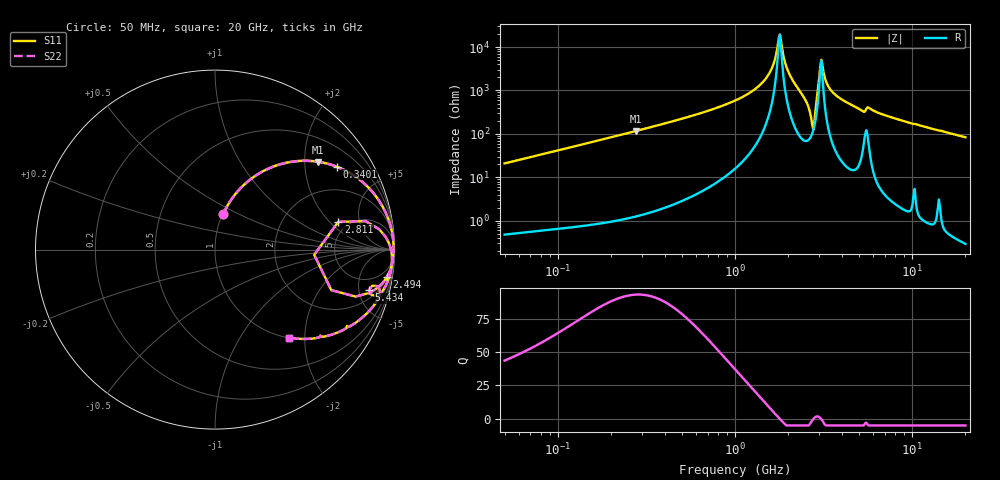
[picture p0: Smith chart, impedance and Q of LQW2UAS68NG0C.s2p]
!Murata Part Number: LQW2UAS68NG0C
!These Parameters are Measured in Series Mode Connection
!  o--[Z]--o
!Port1  Port2
!  o-------o
!Freq. Start=50[MHz] Stop=20[GHz], 401[Steps]
# Hz S RI R 50
!Freq.(Hz) S11(Real) S11(Imag) S21(Real) S21(Imag) S12(Real) S12(Imag) S22(Real) S22(Imag)
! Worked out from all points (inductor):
!   401 points, 50 MHz to 20 GHz, reference 50 ohm
!   read as one part in series: L = 66.3 nH near 51.52 MHz
!   highest Q = 93.1 at 275.8 MHz (marker M1), where L = 67.3 nH
!   self-resonance near 1.767 GHz
!   S11 on the Smith chart (normalised r, x): 50 MHz: 1.01, +0.42; 340.1 MHz: 1.03, +2.91; 2.494 GHz: 2, -12; 2.811 GHz: 4.14, +2.53; 5.434 GHz: 2.98, -6.35; 20 GHz: 1.01, -1.68
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5e7  0.046 0.1983  0.954 -0.1983  0.954 -0.1983  0.046 0.1983
1.364002e8  0.247 0.4247  0.753 -0.4247  0.753 -0.4247  0.247 0.4247
2.757764e8  0.5754 0.4889  0.4246 -0.4889  0.4246 -0.4889  0.5754 0.4889
3.401177e8  0.6773 0.4621  0.3227 -0.4621  0.3227 -0.4621  0.6773 0.4621
3.721004e8  0.7175 0.4447  0.2825 -0.4447  0.2825 -0.4447  0.7175 0.4447
1e9  0.9674 0.1646  0.0326 -0.1646  0.0326 -0.1646  0.9674 0.1646
1.476162e9  0.9923 0.0554  0.00772 -0.0554  0.00772 -0.0554  0.9923 0.0554
1.614971e9  0.9944 0.03  0.00565 -0.03  0.00565 -0.03  0.9944 0.03
1.740566e9  0.995 0.00809  0.00498 -0.00809  0.00498 -0.00809  0.995 0.00809
1.793498e9  0.995 -0.000923  0.00502 0.000923  0.00502 0.000923  0.995 -0.000923
2.021818e9  0.9926 -0.0399  0.00736 0.0399  0.00736 0.0399  0.9926 -0.0399
2.493527e9  0.9575 -0.153  0.0425 0.153  0.0425 0.153  0.9575 -0.153
2.647493e9  0.8623 -0.241  0.1377 0.241  0.1377 0.241  0.8623 -0.241
2.728004e9  0.648 -0.2256  0.352 0.2256  0.352 0.2256  0.648 -0.2256
2.810964e9  0.6867 0.1544  0.3133 -0.1544  0.3133 -0.1544  0.6867 0.1544
3.029571e9  0.9767 0.0143  0.0233 -0.0143  0.0233 -0.0143  0.9767 0.0143
3.121702e9  0.9844 -0.0224  0.0156 0.0224  0.0156 0.0224  0.9844 -0.0224
3.314454e9  0.986 -0.069  0.014 0.069  0.014 0.069  0.986 -0.069
3.626126e9  0.9799 -0.1147  0.0201 0.1147  0.0201 0.1147  0.9799 -0.1147
5.433528e9  0.8584 -0.2262  0.1416 0.2262  0.1416 0.2262  0.8584 -0.2262
7.442007e9  0.8581 -0.3428  0.1419 0.3428  0.1419 0.3428  0.8581 -0.3428
2e10  0.4128 -0.4906  0.5872 0.4906  0.5872 0.4906  0.4128 -0.4906
